DATA_BLOCK "SET POINT-UNIOP"
VERSION : 0.1


  STRUCT
   TEMP_PRERISC_V250 : DWORD ;
   TEMP_MAND_CDZ250 : DWORD ;
   UMID_RIPRESA_LOC : DWORD ;
   TEMP_RIPRESA_LOC_346 : DWORD ;
   TEMP_RIPRESA_LOC_348 : DWORD ;
   TEMP_RIPRESA_LOCALI : DWORD ;
   TEMP_ARIA_EST_CDZ260 : DWORD ;
   TEMP_PRETR_EST_CDZ260 : DWORD ;
   TEMP_RAFFR_CDZ260 : DWORD ;
   TEMP_MANDATA_CDZ260 : DWORD ;
   TEMP_MAND_CDZ380 : DWORD ;
   PRESS_MAND_CDZ380 : DWORD ;
   TEMP_MAND_CDZ390 : DWORD ;
   PRESS_MAND_CDZ390 : DWORD ;
   TEMP_MAND_CDZ400 : DWORD ;
   PRESS_MAND_CDZ400 : DWORD ;
   SOVRA_PRESS_LOC_346 : DWORD ;
   SET_SOVRA_PRESS_LOC_347 : DWORD ;
   SET_SOVRA_PRESS_LOC_346A : DWORD ;
   SET_SOVRA_PRESS_LOC_348 : DWORD ;
   SET_VEL_TUNNEL_BOSCH : DWORD ;
   SET_SOVRA_PRESS_LOC_347A : DWORD ;
   SET_SOVRA_PRESS_LOC_347B : DWORD ;
   SPARE : DWORD ;
   SPARE1 : DWORD ;
   SET_GIRI_INV_250 : DWORD ;
   SET_GIRI_INV_260 : DWORD ;
   SET_GIRI_INV_380 : DWORD ;
   SET_GIRI_INV_390 : DWORD ;
   SET_GIRI_INV_400 : DWORD ;
   SET_TEMPO_GEN_FORMALINA : WORD ;
   SET_TEMPO_ASP_FORMALINA : WORD ;
   SPARE4 : DWORD ;
   SET_APRI_SERRANDE_352 : DWORD ;
   SET_APRI_SERRANDA_355 : DWORD ;
   SET_SERRANDA_HV1236 : DWORD ;
  END_STRUCT ;
BEGIN
   TEMP_PRERISC_V250 := DW#16#41200000;
   TEMP_MAND_CDZ250 := DW#16#41800000;
   UMID_RIPRESA_LOC := DW#16#42200000;
   TEMP_RIPRESA_LOC_346 := DW#16#41B00000;
   TEMP_RIPRESA_LOC_348 := DW#16#41B00000;
   TEMP_RIPRESA_LOCALI := DW#16#41B00000;
   TEMP_ARIA_EST_CDZ260 := DW#16#0;
   TEMP_PRETR_EST_CDZ260 := DW#16#41100000;
   TEMP_RAFFR_CDZ260 := DW#16#41600000;
   TEMP_MANDATA_CDZ260 := DW#16#41A80000;
   TEMP_MAND_CDZ380 := DW#16#41940000;
   PRESS_MAND_CDZ380 := DW#16#42480000;
   TEMP_MAND_CDZ390 := DW#16#41900000;
   PRESS_MAND_CDZ390 := DW#16#41200000;
   TEMP_MAND_CDZ400 := DW#16#41940000;
   PRESS_MAND_CDZ400 := DW#16#0;
   SOVRA_PRESS_LOC_346 := DW#16#22B;
   SET_SOVRA_PRESS_LOC_347 := DW#16#8C;
   SET_SOVRA_PRESS_LOC_346A := DW#16#3C;
   SET_SOVRA_PRESS_LOC_348 := DW#16#0;
   SET_VEL_TUNNEL_BOSCH := DW#16#0;
   SET_SOVRA_PRESS_LOC_347A := DW#16#C8;
   SET_SOVRA_PRESS_LOC_347B := DW#16#0;
   SPARE := DW#16#0;
   SPARE1 := DW#16#0;
   SET_GIRI_INV_250 := DW#16#42BE0000;
   SET_GIRI_INV_260 := DW#16#42480000;
   SET_GIRI_INV_380 := DW#16#42960000;
   SET_GIRI_INV_390 := DW#16#42B40000;
   SET_GIRI_INV_400 := DW#16#42B40000;
   SET_TEMPO_GEN_FORMALINA := W#16#0;
   SET_TEMPO_ASP_FORMALINA := W#16#0;
   SPARE4 := DW#16#0;
   SET_APRI_SERRANDE_352 := DW#16#0;
   SET_APRI_SERRANDA_355 := DW#16#0;
   SET_SERRANDA_HV1236 := DW#16#0;
END_DATA_BLOCK
